(* Logix 5000 AddOnInstructionDefinition export Banner_S15C_MVT_PD_v4; software revision 33.00 *)

TYPE Banner_S15C_MVT_Data_Set_0_v4 :
STRUCT
   Z_Axis_RMS_Velocity : REAL;   // inches per second
   Temperature : REAL;   // F
   X_Axis_RMS_Velocity : REAL;   // inches per second
   Z_Axis_RMS_Peak_Acceleration : REAL;   // G
   X_Axis_RMS_Peak_Acceleration : REAL;   // G
   Z_Axis_Peak_Velocity_Component_Frequency : REAL;   // Hz
   X_Axis_Peak_Velocity_Component_Frequency : REAL;   // Hz
   Z_Axis_Kurtosis : REAL;
   X_Axis_Kurtosis : REAL;
   Z_Axis_Crest_Factor : REAL;
   X_Axis_Crest_Factor : REAL;
   Z_Axis_Peak_Velocity : REAL;   // inches per second
   X_Axis_Peak_Velocity : REAL;   // inches per second
   Z_Axis_High_Frequency_RMS_Acceleration : REAL;   // G
   X_Axis_High_Frequency_RMS_Accleration : REAL;   // G
END_STRUCT
END_TYPE

TYPE Banner_S15C_MVT_Data_Set_1_v4 :
STRUCT
   Z_Axis_RMS_Velocity : REAL;   // mm per second
   Temperature : REAL;   // C
   X_Axis_RMS_Velocity : REAL;   // mm per second
   Z_Axis_RMS_Peak_Acceleration : REAL;   // G
   X_Axis_RMS_Peak_Acceleration : REAL;   // G
   Z_Axis_Peak_Velocity_Component_Frequency : REAL;   // Hz
   X_Axis_Peak_Velocity_Component_Frequency : REAL;   // Hz
   Z_Axis_Kurtosis : REAL;
   X_Axis_Kurtosis : REAL;
   Z_Axis_Crest_Factor : REAL;
   X_Axis_Crest_Factor : REAL;
   Z_Axis_Peak_Velocity : REAL;   // mm per second
   X_Axis_Peak_Velocity : REAL;   // mm per second
   Z_Axis_High_Frequency_RMS_Acceleration : REAL;   // G
   X_Axis_High_Frequency_RMS_Accleration : REAL;   // G
END_STRUCT
END_TYPE

TYPE Banner_S15C_MVT_Data_Set_2_v4 :
STRUCT
   Serial_Number : DINT;
   Model_Number : DINT;
   Production_Date : DINT;
   Firmware_Part_Number : DINT;
   Firmware_Version_Upper : DINT;
   Firmware_Version_Lower : DINT;
   Firmware_Engineering : DINT;
   EEPROM_Part_Number : DINT;
   EEPROM_Version_Upper : DINT;
   EEPROM_Version_Lower : DINT;
END_STRUCT
END_TYPE

TYPE Banner_S15C_MVT_PDIO_v4 :   // UDT with all of the variables needed to control an IO-Link S15C VT.
STRUCT
   Read_Data_Set : SINT;   // 0 = VT English units, 1 = Metric units, 2 = Sensor Information
   Read_Status : SINT;   // 0 = failed, 1 = success
   Counter_Value : INT;
   Data_Set_0 : Banner_S15C_MVT_Data_Set_0_v4;   // English Data Set
   Data_Set_1 : Banner_S15C_MVT_Data_Set_1_v4;   // Metric Data Set
   Data_Set_2 : Banner_S15C_MVT_Data_Set_2_v4;   // Sensor Information Data Set
   DTI : SINT[32];   // Array with Raw Process data being transferred into AOI.
   Write_Data_Set : SINT;   // Set which Data Set should be gathered via the S15C.
END_STRUCT
END_TYPE

ADD_ON_INSTRUCTION Banner_S15C_MVT_PD_v4   (* revision 4.0, vendor Banner Engineering *)
// AOI that used with the S15C MVT sensor.
VAR_IN_OUT
   Process_Data : Banner_S15C_MVT_PDIO_v4; {required}
END_VAR
VAR_INPUT
   Byte_Swap : BOOL; {required}
END_VAR
VAR
   Temp_DWord : DINT[16]; {access None}
   W_Index : SINT; {access None}
   DT_Index : SINT; {access None}
   Data_Update : BOOL; {access None}
END_VAR

ROUTINE Logic   (* ladder *)
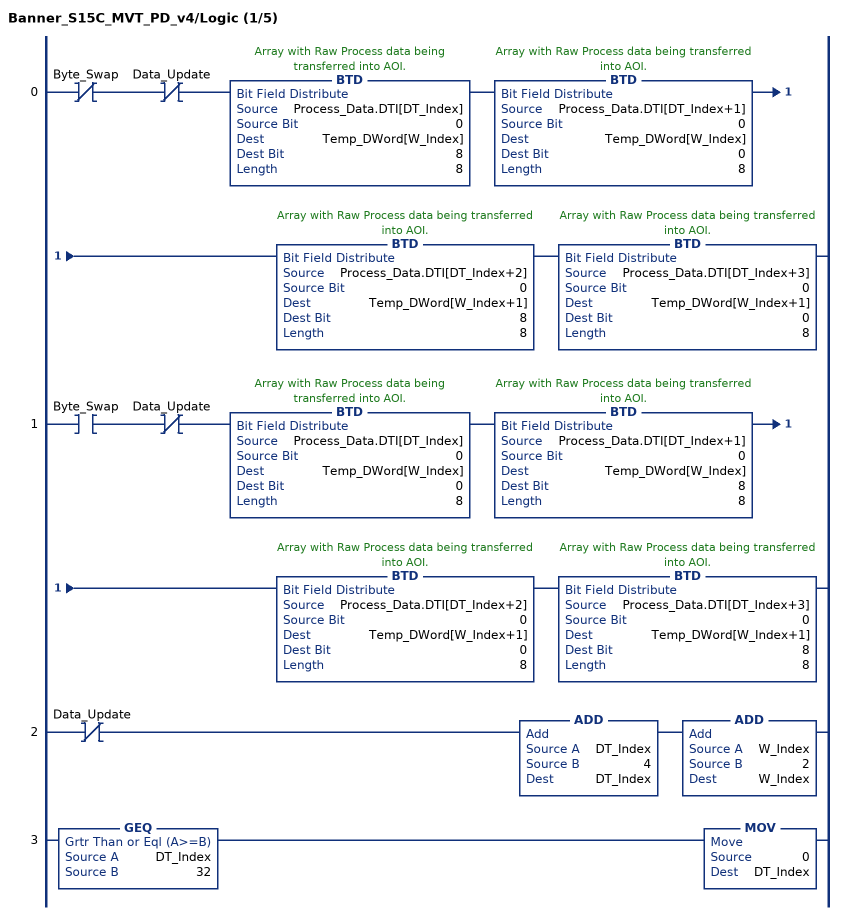
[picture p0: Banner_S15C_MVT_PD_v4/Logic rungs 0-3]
   0: XIO(Byte_Swap)XIO(Data_Update)BTD(Process_Data.DTI[DT_Index],0,Temp_DWord[W_Index],8,8)BTD(Process_Data.DTI[DT_Index+1],0,Temp_DWord[W_Index],0,8)BTD(Process_Data.DTI[DT_Index+2],0,Temp_DWord[W_Index+1],8,8)BTD(Process_Data.DTI[DT_Index+3],0,Temp_DWord[W_Index+1],0,8);
   1: XIC(Byte_Swap)XIO(Data_Update)BTD(Process_Data.DTI[DT_Index],0,Temp_DWord[W_Index],0,8)BTD(Process_Data.DTI[DT_Index+1],0,Temp_DWord[W_Index],8,8)BTD(Process_Data.DTI[DT_Index+2],0,Temp_DWord[W_Index+1],0,8)BTD(Process_Data.DTI[DT_Index+3],0,Temp_DWord[W_Index+1],8,8);
   2: XIO(Data_Update)ADD(DT_Index,4,DT_Index)ADD(W_Index,2,W_Index);
   3: GEQ(DT_Index,32)MOV(0,DT_Index);
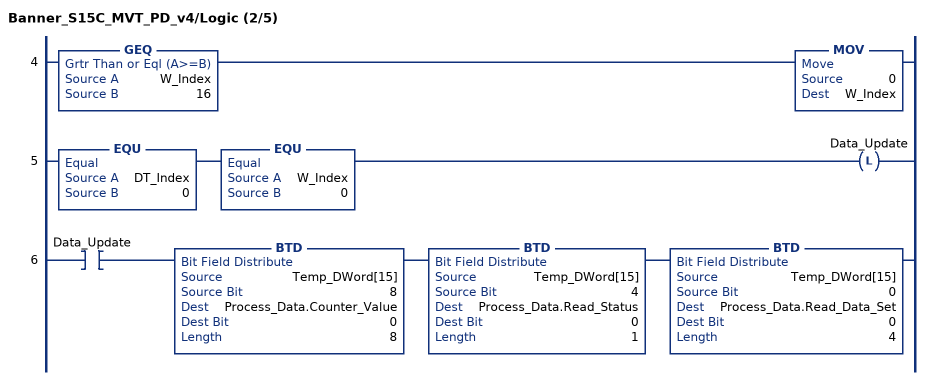
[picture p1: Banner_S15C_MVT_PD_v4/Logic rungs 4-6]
   4: GEQ(W_Index,16)MOV(0,W_Index);
   5: EQU(DT_Index,0)EQU(W_Index,0)OTL(Data_Update);
   6: XIC(Data_Update)BTD(Temp_DWord[15],8,Process_Data.Counter_Value,0,8)BTD(Temp_DWord[15],4,Process_Data.Read_Status,0,1)BTD(Temp_DWord[15],0,Process_Data.Read_Data_Set,0,4);
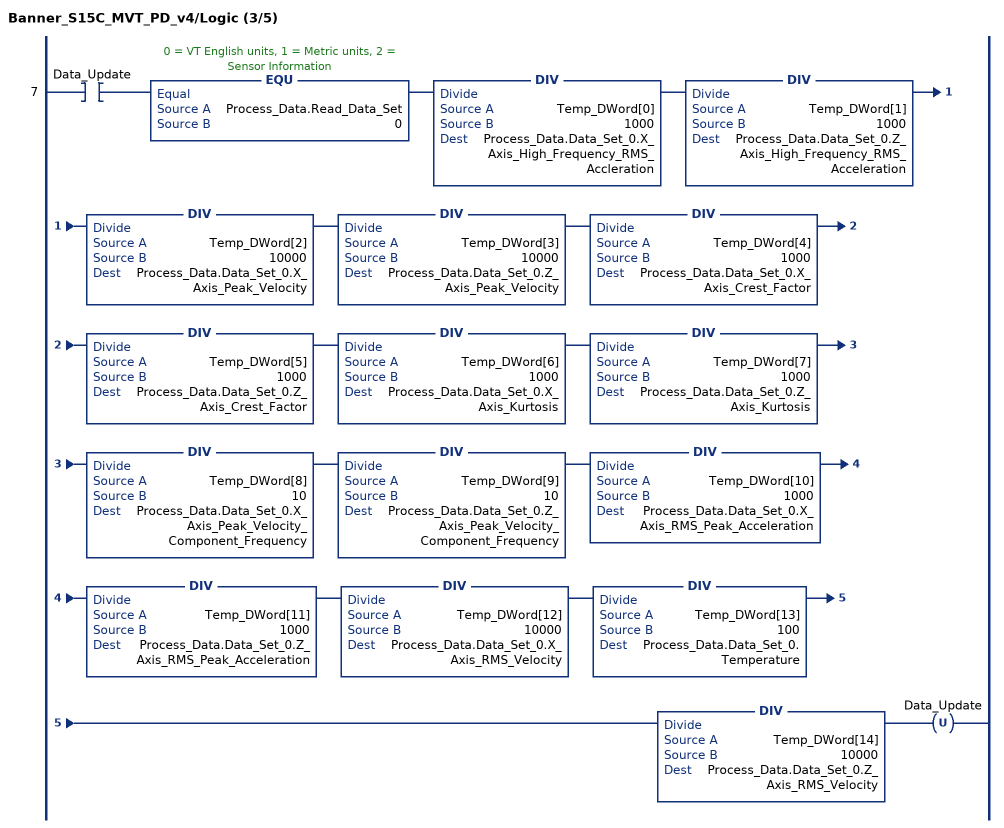
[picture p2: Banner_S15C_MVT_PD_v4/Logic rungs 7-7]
   7: XIC(Data_Update)EQU(Process_Data.Read_Data_Set,0)DIV(Temp_DWord[0],1000,Process_Data.Data_Set_0.X_Axis_High_Frequency_RMS_Accleration)DIV(Temp_DWord[1],1000,Process_Data.Data_Set_0.Z_Axis_High_Frequency_RMS_Acceleration)DIV(Temp_DWord[2],10000,Process_Data.Data_Set_0.X_Axis_Peak_Velocity)DIV(Temp_DWord[3],10000,Process_Data.Data_Set_0.Z_Axis_Peak_Velocity)DIV(Temp_DWord[4],1000,Process_Data.Data_Set_0.X_Axis_Crest_Factor)DIV(Temp_DWord[5],1000,Process_Data.Data_Set_0.Z_Axis_Crest_Factor)DIV(Temp_DWord[6],1000,Process_Data.Data_Set_0.X_Axis_Kurtosis)DIV(Temp_DWord[7],1000,Process_Data.Data_Set_0.Z_Axis_Kurtosis)DIV(Temp_DWord[8],10,Process_Data.Data_Set_0.X_Axis_Peak_Velocity_Component_Frequency)DIV(Temp_DWord[9],10,Process_Data.Data_Set_0.Z_Axis_Peak_Velocity_Component_Frequency)DIV(Temp_DWord[10],1000,Process_Data.Data_Set_0.X_Axis_RMS_Peak_Acceleration)DIV(Temp_DWord[11],1000,Process_Data.Data_Set_0.Z_Axis_RMS_Peak_Acceleration)DIV(Temp_DWord[12],10000,Process_Data.Data_Set_0.X_Axis_RMS_Velocity)DIV(Temp_DWord[13],100,Process_Data.Data_Set_0.Temperature)DIV(Temp_DWord[14],10000,Process_Data.Data_Set_0.Z_Axis_RMS_Velocity)OTU(Data_Update);
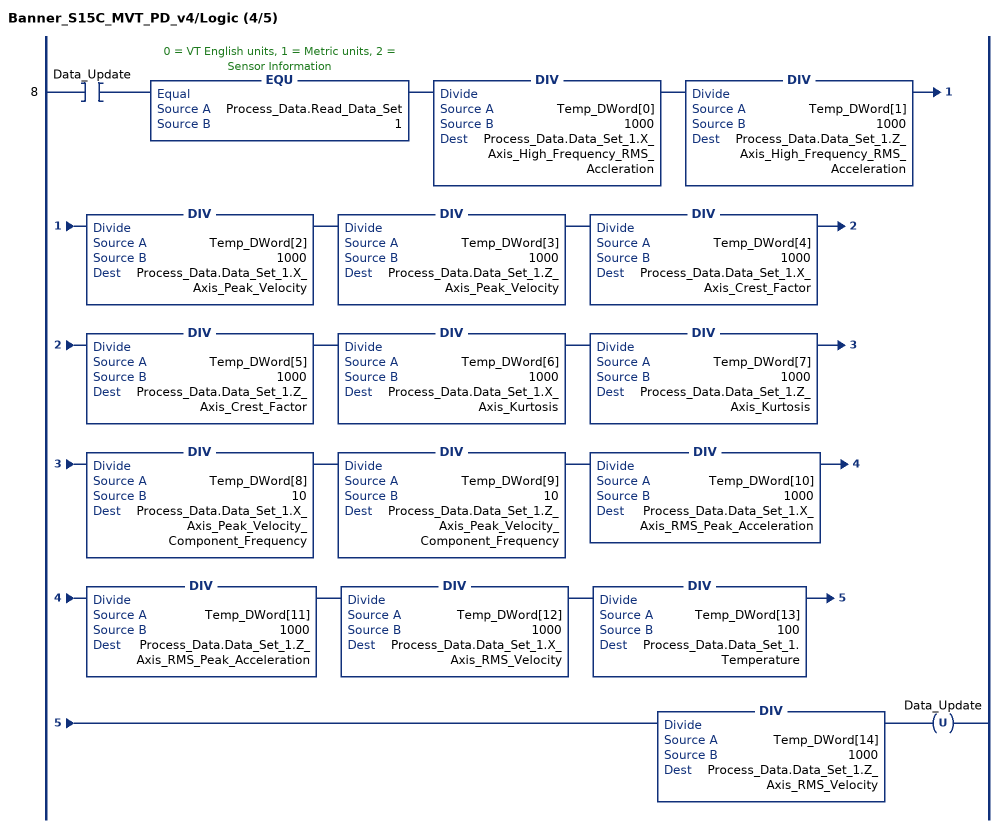
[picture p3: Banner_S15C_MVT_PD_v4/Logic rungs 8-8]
   8: XIC(Data_Update)EQU(Process_Data.Read_Data_Set,1)DIV(Temp_DWord[0],1000,Process_Data.Data_Set_1.X_Axis_High_Frequency_RMS_Accleration)DIV(Temp_DWord[1],1000,Process_Data.Data_Set_1.Z_Axis_High_Frequency_RMS_Acceleration)DIV(Temp_DWord[2],1000,Process_Data.Data_Set_1.X_Axis_Peak_Velocity)DIV(Temp_DWord[3],1000,Process_Data.Data_Set_1.Z_Axis_Peak_Velocity)DIV(Temp_DWord[4],1000,Process_Data.Data_Set_1.X_Axis_Crest_Factor)DIV(Temp_DWord[5],1000,Process_Data.Data_Set_1.Z_Axis_Crest_Factor)DIV(Temp_DWord[6],1000,Process_Data.Data_Set_1.X_Axis_Kurtosis)DIV(Temp_DWord[7],1000,Process_Data.Data_Set_1.Z_Axis_Kurtosis)DIV(Temp_DWord[8],10,Process_Data.Data_Set_1.X_Axis_Peak_Velocity_Component_Frequency)DIV(Temp_DWord[9],10,Process_Data.Data_Set_1.Z_Axis_Peak_Velocity_Component_Frequency)DIV(Temp_DWord[10],1000,Process_Data.Data_Set_1.X_Axis_RMS_Peak_Acceleration)DIV(Temp_DWord[11],1000,Process_Data.Data_Set_1.Z_Axis_RMS_Peak_Acceleration)DIV(Temp_DWord[12],1000,Process_Data.Data_Set_1.X_Axis_RMS_Velocity)DIV(Temp_DWord[13],100,Process_Data.Data_Set_1.Temperature)DIV(Temp_DWord[14],1000,Process_Data.Data_Set_1.Z_Axis_RMS_Velocity)OTU(Data_Update);
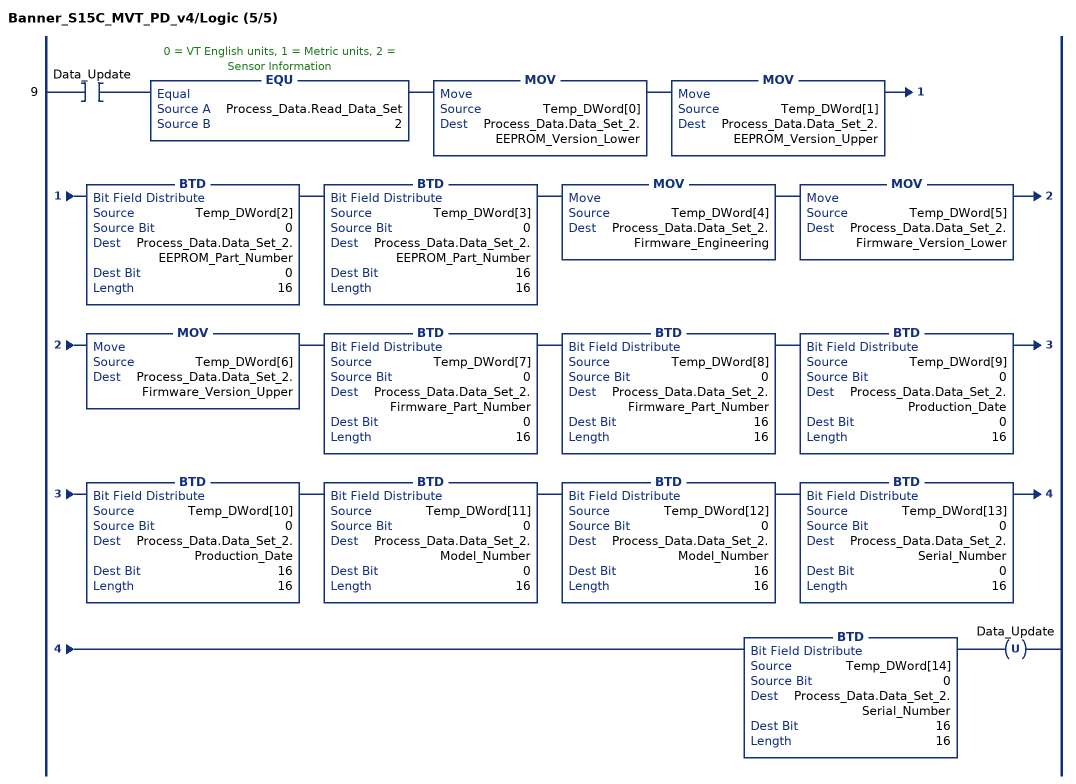
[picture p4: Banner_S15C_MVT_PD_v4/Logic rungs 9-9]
   9: XIC(Data_Update)EQU(Process_Data.Read_Data_Set,2)MOV(Temp_DWord[0],Process_Data.Data_Set_2.EEPROM_Version_Lower)MOV(Temp_DWord[1],Process_Data.Data_Set_2.EEPROM_Version_Upper)BTD(Temp_DWord[2],0,Process_Data.Data_Set_2.EEPROM_Part_Number,0,16)BTD(Temp_DWord[3],0,Process_Data.Data_Set_2.EEPROM_Part_Number,16,16)MOV(Temp_DWord[4],Process_Data.Data_Set_2.Firmware_Engineering)MOV(Temp_DWord[5],Process_Data.Data_Set_2.Firmware_Version_Lower)MOV(Temp_DWord[6],Process_Data.Data_Set_2.Firmware_Version_Upper)BTD(Temp_DWord[7],0,Process_Data.Data_Set_2.Firmware_Part_Number,0,16)BTD(Temp_DWord[8],0,Process_Data.Data_Set_2.Firmware_Part_Number,16,16)BTD(Temp_DWord[9],0,Process_Data.Data_Set_2.Production_Date,0,16)BTD(Temp_DWord[10],0,Process_Data.Data_Set_2.Production_Date,16,16)BTD(Temp_DWord[11],0,Process_Data.Data_Set_2.Model_Number,0,16)BTD(Temp_DWord[12],0,Process_Data.Data_Set_2.Model_Number,16,16)BTD(Temp_DWord[13],0,Process_Data.Data_Set_2.Serial_Number,0,16)BTD(Temp_DWord[14],0,Process_Data.Data_Set_2.Serial_Number,16,16)OTU(Data_Update);
END_ROUTINE
END_ADD_ON_INSTRUCTION
